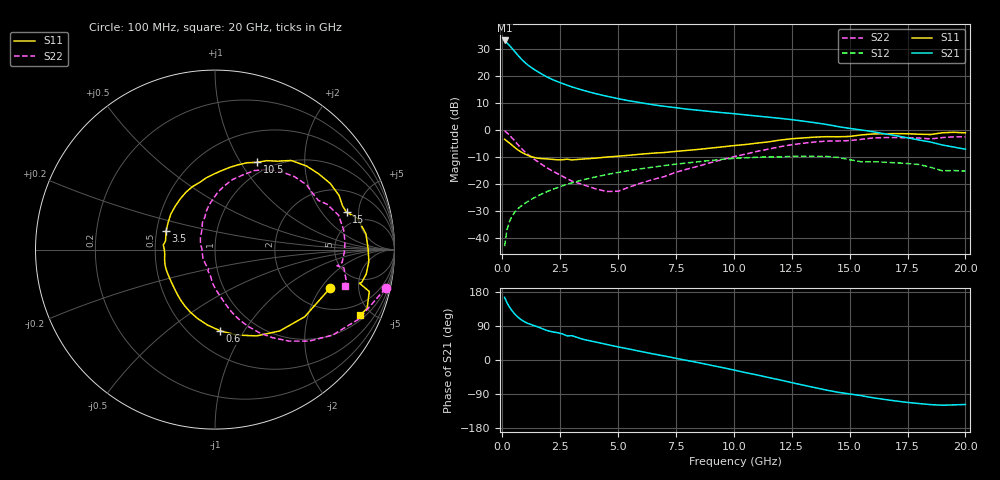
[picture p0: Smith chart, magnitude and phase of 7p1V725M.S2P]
! Infineon Technologies  Discrete & RF Semiconductors
! bfp620
! VCE =  1.7 V,  IC =  25 mA
! Common Emitter S-Parameters:  Sep 2002
# GHz  S  MA  R  50
!  f  S11  S21  S12  S22
! GHz  MAG  ANG  MAG  ANG  MAG  ANG  MAG  ANG
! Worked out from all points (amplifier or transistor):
!   59 points, 100 MHz to 20 GHz, reference 50 ohm
!   highest |S21| = 33.2 dB at 100 MHz (marker M1)
!   |S21| within 3 dB of that: start of sweep to 428 MHz
!   unconditionally stable (mu >= 1): 3.166 GHz to 9.908 GHz; 17.16 GHz to end of sweep
!   at 1 GHz: K = 0.73, MSG = 25.9 dB, |S12| = -27.0 dB
!   at 5.5 GHz: K = 1.04, MAG = 11.7 dB, |S12| = -15.0 dB
!   at 20 GHz: K = 1.30, MAG = 0.8 dB, |S12| = -15.2 dB
!   S11 on the Smith chart (normalised r, x): 100 MHz: 3.08, -2.45; 600 MHz: 0.69, -0.79; 3.5 GHz: 0.56, +0.13; 10.5 GHz: 0.86, +1.18; 15 GHz: 3.67, +3.63; 20 GHz: 1.25, -4.32
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0.1  0.6751 -18.7  45.5 165.3  0.0071 76.5  0.9743 -12.8
0.2  0.6244 -36.8  41.02 151.5  0.0141 73.0  0.8896 -25.8
0.3  0.5791 -51.5  37.06 140.6  0.0198 69.2  0.8103 -36.0
0.4  0.534 -64.2  33.26 131.6  0.0246 66.0  0.7313 -44.2
0.5  0.4913 -75.7  29.67 124.0  0.0287 63.4  0.655 -51.1
0.6  0.4536 -86.3  26.41 117.4  0.0323 61.5  0.5846 -57.0
0.7  0.4219 -95.8  23.55 111.8  0.0357 60.0  0.5223 -62.1
0.8  0.3956 -104.3  21.13 106.9  0.0388 59.0  0.4689 -66.4
0.9  0.374 -111.8  19.11 102.9  0.0418 58.3  0.424 -70.0
1.1  0.3406 -124.0  16.07 96.8  0.0476 57.5  0.3552 -75.4
1.3  0.3175 -134.0  13.92 92.3  0.0535 56.8  0.3053 -79.3
1.8  0.2946 -155.6  10.31 80.9  0.0685 54.6  0.2173 -89.4
2.2  0.2861 -169.1  8.476 73.8  0.0807 52.4  0.1715 -96.3
2.8  0.2891 175.0  6.757 63.5  0.099 48.2  0.1251 -108.5
3.5  0.2911 159.5  5.426 54.4  0.1204 42.5  0.0971 -122.5
5  0.3284 132.3  3.813 34.6  0.1643 29.1  0.0737 174.7
7  0.3843 102.7  2.749 10.6  0.22 10.4  0.1379 121.0
10.5  0.5397 64.3  1.909 -33.3  0.3072 -28.6  0.3591 81.6
13.5  0.7402 29.9  1.368 -72.9  0.3254 -64.5  0.6013 42.5
15  0.7621 15.8  1.072 -89.6  0.2833 -85.5  0.6381 25.4
17  0.8598 -4.5  0.789 -108.2  0.2477 -96.1  0.7257 3.4
20  0.8882 -24.2  0.442 -117.4  0.1742 -106.2  0.7517 -15.7
